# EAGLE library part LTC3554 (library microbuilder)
LTC3554 - USB Power Manager with Li-Ion Charger and Two Step-Down Regulators The LTC3554 is a micropower, highly integrated power management and battery charger IC for single-cell Li-Ion/Polymer battery applications. The LTC3554 also includes two synchronous step-down switching regulators as well as a pushbutton controller.
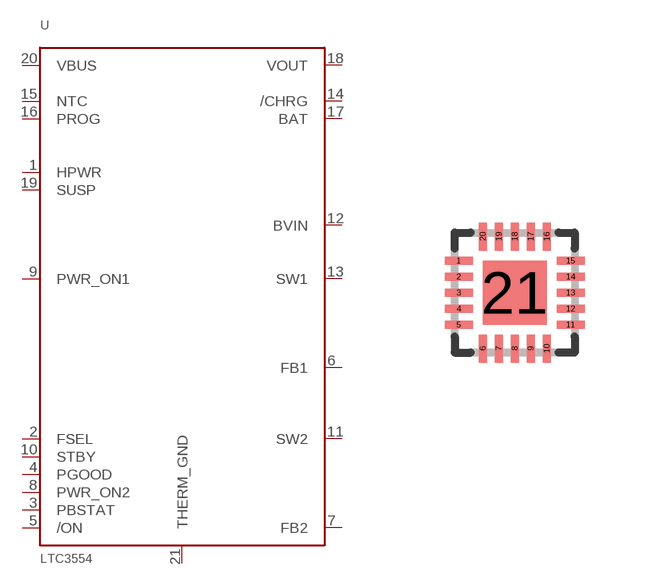
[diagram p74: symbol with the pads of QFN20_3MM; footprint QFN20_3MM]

Designator prefix U

## LTC3554  [QFN20_3MM]
1  HPWR
2  FSEL
3  PBSTAT
4  PGOOD
5  /ON
6  FB1
7  FB2
8  PWR_ON2
9  PWR_ON1
10  STBY
11  SW2
12  BVIN
13  SW1
14  /CHRG
15  NTC
16  PROG
17  BAT
18  VOUT
19  SUSP
20  VBUS
21  THERM_GND

## Footprint QFN20_3MM (pad centres in mm)
20-Lead Plastic QFN (3mm x 3mm, 20-pin 0.4mm pitch) Source: http://cds.linear.com/docs/Datasheet/3554fa.pdf
smd 0.7 x 0.2: 1 -1.4,0.8; 2 -1.4,0.4; 3 -1.4,0; 4 -1.4,-0.4; 5 -1.4,-0.8; 11 1.4,-0.8; 12 1.4,-0.4; 13 1.4,0; 14 1.4,0.4; 15 1.4,0.8
smd 0.2 x 0.7: 6 -0.8,-1.4; 7 -0.4,-1.4; 8 0,-1.4; 9 0.4,-1.4; 10 0.8,-1.4; 16 0.8,1.4; 17 0.4,1.4; 18 0,1.4; 19 -0.4,1.4; 20 -0.8,1.4
smd 1.6 x 1.6: 21 0,0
